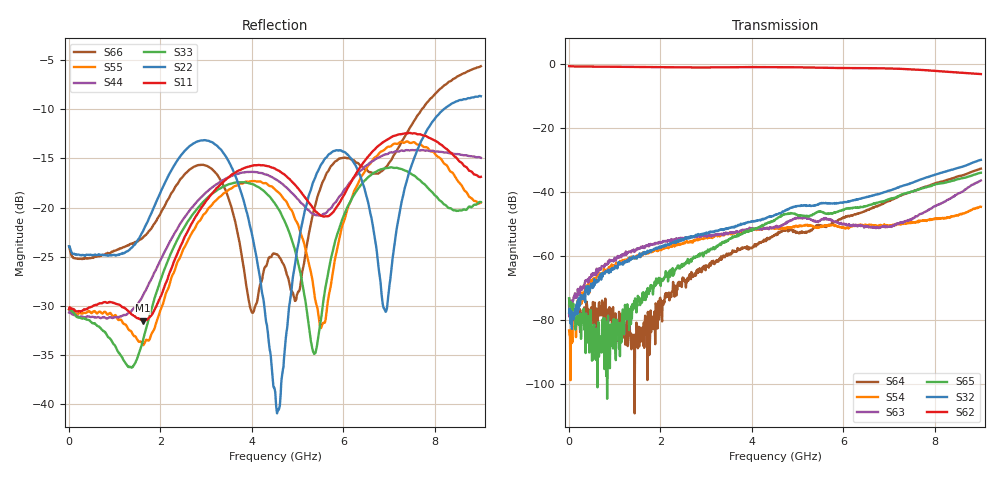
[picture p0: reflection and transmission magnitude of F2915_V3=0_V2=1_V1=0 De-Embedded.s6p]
! Integrated Device Technology
! Corporate Headquarters
! 6024 Silver Creek Valley Road
! San Jose, CA 95138  USA
! Phone:  1-408-284-8200
! Toll Free:  1-800-223-1366
! Webpage:  http://www.idt.com/
! Timing and RF Division
! 515 Groton Road, Suite 102
! Westford, MA 01886-6024
! Device:  F2915
! Description: High Reliability SP5T RF Switch
! Frequency:  0.05 -  8.GHz
! Package:  4x4 mm Thin QFN Plastic Package: 24 pin
! Ports:  6 RF,  5 DC
!  Pin  1  = GND
!  Pin  2  = RF5  =  Port 5
!  Pin  3  = GND
!  Pin  4  = GND
!  Pin  5  = RF4  =  Port 4
!  Pin  6  = GND
!  Pin  7  = GND
!  Pin  8  = RF3  =  Port 3
!  Pin  9  = GND
!  Pin 10  = GND
!  Pin 11  = RF2  =  Port 2
!  Pin 12  = GND
!  Pin 13  = GND
!  Pin 14  = RF1  =  Port 1
!  Pin 15  = GND
!  Pin 16  = Vcc
!  Pin 17  = V1
!  Pin 18  = V2
!  Pin 19  = V3
!  Pin 20  = VSSext
!  Pin 21  = GND
!  Pin 22  = RFC  =  Port 6
!  Pin 23  = GND
!  Pin 24  = GND
! Voltage:  VDD  =  +3.30 Volts
!  VSSEXT =  0.00 Volts
! Current:  IDD  = 253  uA
! State:  RF2 Selected
! V1:  Logic LOW
! V2:  Logic HIGH
! V3:  Logic LOW
! Data:  The device was measured on the F291x evaluation board which has
!  individual transmission lines to the RF pins.  Data was collected
!  using a calibrated network analyzer.  The input lines were
!  modeled using Automatic Fixture Removal (AFR) from Keysight.
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# Hz S  dB  R 50
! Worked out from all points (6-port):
!   900 points, 10 MHz to 9 GHz, reference 50 ohm
!   strongest paths, dB at 10 MHz, 2.26 GHz, 4.51 GHz, 6.76 GHz, 9 GHz:
!     S62: -0.8, -1.1, -1.1, -1.4, -3.2
!     S32: -77.8, -56.0, -47.3, -40.8, -30.0
!     S65: -73.3, -65.6, -48.7, -43.3, -34.1
!     S63: -75.4, -55.3, -51.0, -51.3, -36.5
!     S54: -83.3, -56.8, -51.6, -50.8, -44.7
!     S64: -73.3, -71.2, -53.3, -44.3, -32.8
!   lowest |S11| = -31.5 dB at 1.62 GHz (marker M1), VSWR 1.05, Z = 49.5 + j2.61 ohm
!   |S11| at or under -10 dB: start of sweep to end of sweep
